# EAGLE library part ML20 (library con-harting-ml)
HARTING
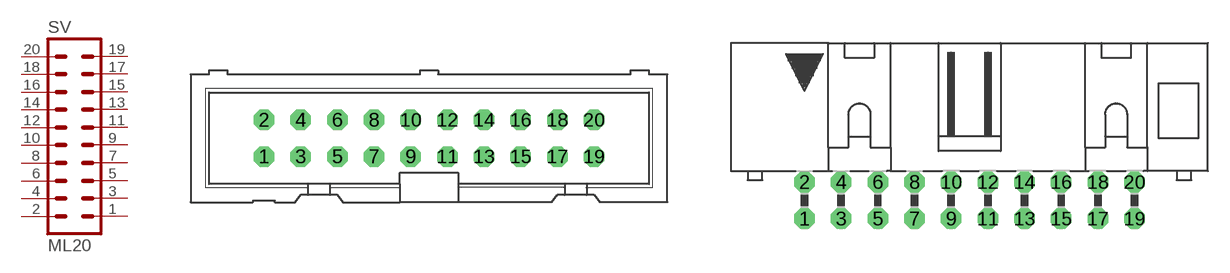
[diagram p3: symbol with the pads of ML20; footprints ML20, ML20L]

Designator prefix SV

## ML20 (OC_FARNELL: unknown; OC_NEWARK: unknown)  [ML20]
1  1  pas
2  2  pas
3  3  pas
4  4  pas
5  5  pas
6  6  pas
7  7  pas
8  8  pas
9  9  pas
10  10  pas
11  11  pas
12  12  pas
13  13  pas
14  14  pas
15  15  pas
16  16  pas
17  17  pas
18  18  pas
19  19  pas
20  20  pas

## ML20L (OC_FARNELL: unknown; OC_NEWARK: unknown)  [ML20L]
Pads as for ML20

## ML203M (OC_FARNELL: unknown; OC_NEWARK: unknown)  [3M_20]
Pads as for ML20

## ML203ML (OC_FARNELL: unknown; OC_NEWARK: unknown)  [3M_20L]
Pads as for ML20

## Footprint ML20 (pad centres in mm)
HARTING
drill 0.914 octagon: 1 -11.43,-1.27; 2 -11.43,1.27; 3 -8.89,-1.27; 4 -8.89,1.27; 5 -6.35,-1.27; 6 -6.35,1.27; 7 -3.81,-1.27; 8 -3.81,1.27; 9 -1.27,-1.27; 10 -1.27,1.27; 11 1.27,-1.27; 12 1.27,1.27; 13 3.81,-1.27; 14 3.81,1.27; 15 6.35,-1.27; 16 6.35,1.27; 17 8.89,-1.27; 18 8.89,1.27; 19 11.43,-1.27; 20 11.43,1.27

## Footprint ML20L (pad centres in mm)
HARTING
drill 0.914 octagon: 1 -11.43,-1.27; 2 -11.43,1.27; 3 -8.89,-1.27; 4 -8.89,1.27; 5 -6.35,-1.27; 6 -6.35,1.27; 7 -3.81,-1.27; 8 -3.81,1.27; 9 -1.27,-1.27; 10 -1.27,1.27; 11 1.27,-1.27; 12 1.27,1.27; 13 3.81,-1.27; 14 3.81,1.27; 15 6.35,-1.27; 16 6.35,1.27; 17 8.89,-1.27; 18 8.89,1.27; 19 11.43,-1.27; 20 11.43,1.27

## Footprint 3M_20 (pad centres in mm)
3M
drill 0.813 square: 1 -11.43,-1.27; 2 -11.43,1.27; 3 -8.89,-1.27; 4 -8.89,1.27; 5 -6.35,-1.27; 6 -6.35,1.27; 7 -3.81,-1.27; 8 -3.81,1.27; 9 -1.27,-1.27; 10 -1.27,1.27; 11 1.27,-1.27; 12 1.27,1.27; 13 3.81,-1.27; 14 3.81,1.27; 15 6.35,-1.27; 16 6.35,1.27; 17 8.89,-1.27; 18 8.89,1.27; 19 11.43,-1.27; 20 11.43,1.27

## Footprint 3M_20L (pad centres in mm)
3M
drill 0.813 square: 1 -11.43,-5.08; 2 -11.43,-2.54; 3 -8.89,-5.08; 4 -8.89,-2.54; 5 -6.35,-5.08; 6 -6.35,-2.54; 7 -3.81,-5.08; 8 -3.81,-2.54; 9 -1.27,-5.08; 10 -1.27,-2.54; 11 1.27,-5.08; 12 1.27,-2.54; 13 3.81,-5.08; 14 3.81,-2.54; 15 6.35,-5.08; 16 6.35,-2.54; 17 8.89,-5.08; 18 8.89,-2.54; 19 11.43,-5.08; 20 11.43,-2.54
hole 2.54 at -17.348,-3.277
hole 2.54 at 17.348,-3.277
